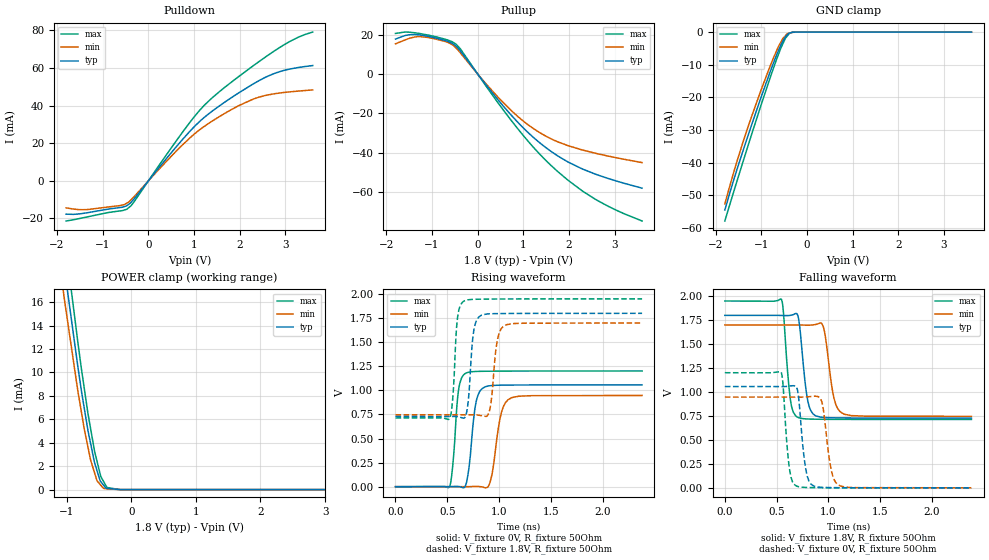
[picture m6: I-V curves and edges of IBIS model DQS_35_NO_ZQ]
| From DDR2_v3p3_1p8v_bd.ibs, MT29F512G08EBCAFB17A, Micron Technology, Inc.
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| MODEL DQS_35_NO_ZQ (35 Ohm Data Strobe I/O with no ODT, With No Cal)
[Model]   DQS_35_NO_ZQ
Model_type   I/O
Vinl = 650.000mV
Vinh = 1.150V
Vmeas = 900.000mV
Vref = 900.000mV
Cref = 0.0pF
Rref = 50.000Ohm
|   typ   min   max
|C_comp   1.200pF   1.100pF   1.300pF
C_comp_pullup   0.6000pF   0.5500pF   0.6500pF
C_comp_pulldown   0.6000pF   0.5500pF   0.6500pF
[Model Spec]
| Input threshold voltage corners
Vinl   0.6500V   0.6000V   0.7250V
Vinh   1.1500V   1.1000V   1.2250V
| Measurement voltage corners
Vmeas   0.9000V   0.8500V   0.9750V
| Timing spec test load voltage corners
Vref   0.9000V   0.8500V   0.9750V
| Dynamic Overshoot Parameters from ONFI4 Specification
D_overshoot_ampl_h   1.00   NA   NA
D_overshoot_ampl_l   1.00   NA   NA
D_overshoot_area_h   0.75n   NA   NA
D_overshoot_area_l   0.75n   NA   NA
[Receiver Thresholds]
|Vth   =  0.900V
|Vth_min  =  0.8820V
|Vth_max  =  0.9180V
|Vinh_ac  =  0.250V
|Vinh_dc  =  0.125V
|Vinl_ac  = -0.250V
|Vinl_dc  = -0.125V
|Tslew_ac =  5.000ns |Not specified, so set to high value
|Threshold_sensitivity = 0.50
|Reference_supply Pullup_ref
Vcross_low   = 0.725V
Vcross_high  = 1.075V
Vdiff_ac   = 500mV
Vdiff_dc   = 250mV
Tdiffslew_ac = 10.000ns |Not specified, so set to high value
[Voltage Range]   1.8000V   1.7000V   1.9500V
[Pullup Reference]   1.8000V   1.7000V   1.9500V
| Junction Temperature (Ambient temp is 35C typ, 70C min, 0C max)
[Temperature Range]   50.0   85.0   0.0
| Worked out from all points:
|   slope of the pulldown table from 0 to 0.27 V, typ, clamps not added: 33.1 ohm
|   slope of the pullup table from 0 to 0.27 V, typ, clamps not added: 33.4 ohm
|   GND clamp passes 1 mA (typ) near -0.44 V on its own axis
|   POWER clamp passes 1 mA (typ) near -0.50 V on its own axis
|   falling waveform, V_fixture 1.8V, R_fixture 50Ohm: 20-80 % time 62.7ps typ, 74.2ps min, 53.7ps max; typ from 1.8 V to 0.728 V
|   rising waveform, V_fixture 0V, R_fixture 50Ohm: 20-80 % time 61.4ps typ, 78.4ps min, 49.4ps max; typ from 0 V to 1.06 V
|   rising waveform, V_fixture 1.8V, R_fixture 50Ohm: 20-80 % time 44.4ps typ, 52.3ps min, 38ps max; typ from 0.728 V to 1.8 V
|   falling waveform, V_fixture 0V, R_fixture 50Ohm: 20-80 % time 58ps typ, 68.5ps min, 50.1ps max; typ from 1.06 V to 0 V
[Pulldown]
|   Voltage   I(typ)   I(min)   I(max)
-1.8V     -17.7mA    -14.36mA   -21.34mA
-1.331V   -16.91mA   -15.24mA   -19.12mA
-630.4mV  -14.2mA    -13.16mA   -15.98mA
-473.4mV  -13.2mA    -11.88mA   -15.08mA
-313.2mV  -9.601mA   -8.423mA   -11.12mA
776mV     22.77mA    19.79mA    26.8mA
1.116V    31.44mA    27.04mA    37.31mA
1.394V    37.03mA    31.74mA    44.1mA
1.985V    46.91mA    40.09mA    55.61mA
2.614V    55.67mA    45.71mA    66.71mA
3.092V    59.47mA    47.35mA    74.09mA
3.6V      61.35mA    48.4mA     79.18mA
[GND Clamp]
|   Voltage   I(typ)   I(min)   I(max)
-1.8V     -54.56mA   -52.69mA   -57.93mA
-1.554V   -43.01mA   -40.54mA   -46.59mA
-1.336V   -33.61mA   -30.93mA   -36.81mA
-1.036V   -21.2mA    -18.93mA   -23.66mA
-829.3mV  -13.08mA   -11.23mA   -14.95mA
-630.4mV  -5.889mA   -4.612mA   -7.067mA
-531.8mV  -2.931mA   -2.046mA   -3.69mA
-472.1mV  -1.487mA   -1.111mA   -1.902mA
-431.5mV  -903.3uA   -483.2uA   -1.222mA
-378mV    -285.6uA   -293uA     -327uA
-178.2mV  -2.719uA   -1.561uA   -751.9nA
3.604V    0A         0A         0A
[Pullup]
|   Voltage   I(typ)   I(min)   I(max)
-1.8V     17.84mA    15.4mA     20.68mA
-1.492V   20.03mA    18.23mA    21.32mA
-1.242V   19.84mA    19.05mA    20.53mA
-729mV    17.17mA    16.69mA    17.85mA
-472.1mV  14.17mA    13.21mA    15.18mA
564.7mV   -16.42mA   -14.66mA   -18.41mA
957.4mV   -26.46mA   -23.16mA   -30.13mA
1.359V    -35mA      -29.83mA   -40.79mA
1.765V    -41.86mA   -34.62mA   -49.89mA
2.301V    -48.43mA   -38.72mA   -59.68mA
2.866V    -53.25mA   -41.82mA   -67.44mA
3.6V      -58.12mA   -45.09mA   -74.85mA
[POWER Clamp]
|   Voltage   I(typ)   I(min)   I(max)
-1.8V     59.37mA    57.52mA    61.9mA
-1.055V   19.69mA    17mA       22.54mA
-1.034V   18.79mA    16.14mA    21.56mA
-829.3mV  10.55mA    8.462mA    12.64mA
-729mV    6.964mA    5.185mA    8.66mA
-630.4mV  3.937mA    2.522mA    5.201mA
-531mV    1.618mA    753.4uA    2.409mA
-472.1mV  669.5uA    367.5uA    1.103mA
-431.5mV  391.1uA    106.3uA    708.2uA
-376.5mV  100.3uA    62.6uA     180.1uA
-178.2mV  0A         501.6nA    561.5nA
3.604V    0A         0A         0A
[Ramp]
R_load = 50
|   typ   min   max
dV/dt_r 6.3425E-01/6.1156E-11   5.6816E-01/7.7489E-11   7.2087E-01/4.9145E-11
dV/dt_f 6.4316E-01/6.2537E-11   5.7228E-01/7.3865E-11   7.4183E-01/5.3549E-11
[Falling Waveform]
V_fixture = 1.8V
V_fixture_min = 1.7V
V_fixture_max = 1.95V
R_fixture = 50Ohm
C_fixture = 0F
|   Time   V(typ)   V(min)   V(max)
0s        1.8V       1.7V       1.95V
546ps     1.799V     1.7V       1.969V
634ps     1.801V     1.7V       911.8mV
706ps     1.793V     1.7V       735.2mV
792ps     960.4mV    1.698V     719.1mV
870ps     756.6mV    1.704V     716.6mV
950ps     735.4mV    1.684V     715.5mV
1.052ns   730.9mV    943.2mV    714.8mV
1.15ns    729.7mV    769.2mV    714.4mV
2.38ns    728.1mV    746.1mV    713.6mV
[Rising Waveform]
V_fixture = 0V
V_fixture_min = 0V
V_fixture_max = 0V
R_fixture = 50Ohm
C_fixture = 0F
|   Time   V(typ)   V(min)   V(max)
0s        77.71uV    151uV      22.52uV
520ps     407uV      107.6uV    -4.55mV
552ps     1.505mV    105uV      213.2mV
608ps     1.597mV    70.13uV    998.6mV
684ps     38.38mV    162.8uV    1.181V
778ps     879.3mV    2.272mV    1.196V
866ps     1.037V     -11.36mV   1.198V
922ps     1.049V     81.9mV     1.199V
1.086ns   1.055V     902.5mV    1.2V
2.38ns    1.057V     947.1mV    1.201V
[Rising Waveform]
V_fixture = 1.8V
V_fixture_min = 1.7V
V_fixture_max = 1.95V
R_fixture = 50Ohm
C_fixture = 0F
|   Time   V(typ)   V(min)   V(max)
0s        728mV      746mV      713.6mV
522ps     728.3mV    746mV      704.2mV
600ps     726.8mV    745.9mV    1.764V
666ps     715.3mV    745.9mV    1.93V
756ps     1.623V     746.3mV    1.945V
830ps     1.78V      737.5mV    1.947V
904ps     1.794V     774.2mV    1.948V
984ps     1.797V     1.527V     1.948V
1.068ns   1.798V     1.681V     1.949V
2.38ns    1.8V       1.7V       1.95V
[Falling Waveform]
|Gnd
V_fixture = 0V
V_fixture_min = 0V
V_fixture_max = 0V
R_fixture = 50Ohm
C_fixture = 0F
|   Time   V(typ)   V(min)   V(max)
0s        1.057V     947.2mV    1.201V
542ps     1.056V     947.3mV    1.209V
624ps     1.062V     947.3mV    198.2mV
692ps     1.05V      946.9mV    19.04mV
782ps     191.3mV    948.4mV    4.38mV
856ps     20.36mV    956.1mV    2.688mV
936ps     4.976mV    897.5mV    1.813mV
1.024ns   2.434mV    204.2mV    1.316mV
1.088ns   1.772mV    35.8mV     1.078mV
2.38ns    156.7uV    268.8uV    64.47uV
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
